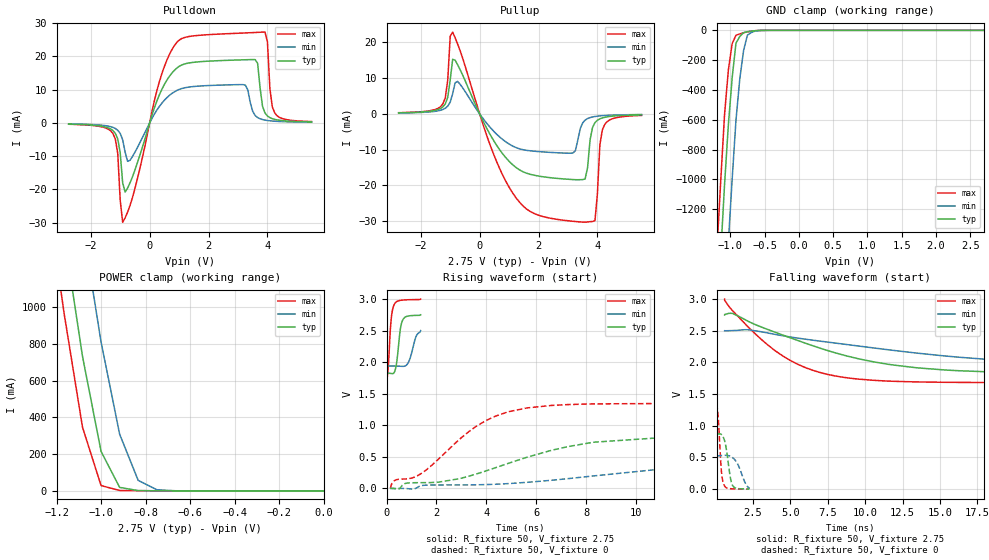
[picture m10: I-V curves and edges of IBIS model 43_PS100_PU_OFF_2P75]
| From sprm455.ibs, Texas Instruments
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|   Model Cell 43_PS100_PU_OFF_2P75
|IDG09_OUO43_PS100_PU_OFF_2P75
[Model]   43_PS100_PU_OFF_2P75
Model_type   I/O
Polarity   Non-Inverting
Enable   Active-Low
Vinl =  0.7V
Vinh =  1.7V
Cref =  15pF
Rref =  100.00M
Vref =  0V
Vmeas =  1.375
C_comp   1.5660002p   1.4978002p   1.7490998p
[Model Spec]
Vinl   0.7V   0.7V   0.7V
Vinh   1.7V   1.7V   1.7V
[Temperature Range]   25   125   -40
[Voltage Range]   2.75   2.5   3
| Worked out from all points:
|   slope of the pulldown table from 0 to 0.412 V, typ, clamps not added: 41 ohm
|   slope of the pullup table from 0 to 0.412 V, typ, clamps not added: 62.6 ohm
|   GND clamp passes 1 mA (typ) near -0.58 V on its own axis
|   POWER clamp passes 1 mA (typ) near -0.78 V on its own axis
|   rising waveform, R_fixture 50, V_fixture 2.75: 20-80 % time 161ps typ, 231ps min, 130ps max; typ from 1.82 V to 2.75 V
|   rising waveform, R_fixture 50, V_fixture 0: 20-80 % time 4.57ns typ, 8.78ns min, 2.5ns max; typ from 0 V to 0.861 V
|   falling waveform, R_fixture 50, V_fixture 2.75: 20-80 % time 7.55ns typ, 12.6ns min, 4.28ns max; typ from 2.75 V to 1.82 V
|   falling waveform, R_fixture 50, V_fixture 0: 20-80 % time 319ps typ, 552ps min, 204ps max; typ from 0.861 V to 0 V
[POWER_clamp]
|   voltage   I(typ)   I(min)   I(max)
-2.75V    16.6A      17.26A     16.24A
-1.194V   1.641A     2.388A     1.212A
-1.167V   1.399A     2.143A     971.7mA
-1.139V   1.177A     1.911A     763.3mA
-1.111V   954.8mA    1.678A     555mA
-1.083V   732.5mA    1.445A     346.6mA
-1.056V   560.1mA    1.234A     240.8mA
-1.028V   387.7mA    1.022A     135mA
-1V       215.3mA    810.7mA    29.13mA
-916.7mV  19.33mA    309.1mA    2.488mA
-833.3mV  1.75mA     57.46mA    1.352mA
0V        27.64pA    4.396nA    364.2fA
[Pulldown]
|   voltage   I(typ)   I(min)   I(max)
-2.75V    -365.9uA   -284.1uA   -404.8uA
-1.25V    -2.274mA   -1.347mA   -3.141mA
-1.083V   -4.807mA   -2.213mA   -9.196mA
-916.7mV  -18.05mA   -5.07mA    -29.89mA
-666.7mV  -18.05mA   -11.25mA   -24.87mA
333.3mV   8.511mA    4.998mA    12.5mA
1.083V    17.41mA    10.32mA    25.36mA
3.25V     19.01mA    11.37mA    27.08mA
3.583V    19.04mA    2.232mA    27.22mA
3.917V    2.992mA    841.3uA    27.33mA
4.25V     1.053mA    505.4uA    2.946mA
5.5V      292.8uA    198.8uA    397.1uA
[Pullup]
|   voltage   I(typ)   I(min)   I(max)
-2.75V    285.7uA    234.9uA    326.2uA
-1.25V    1.953mA    1.223mA    2.77mA
-1.083V   4.622mA    2.158mA    9.493mA
-916.7mV  15.25mA    5.649mA    22.87mA
-750mV    13.77mA    9.085mA    19.58mA
1.167V    -14.54mA   -9.171mA   -22.68mA
3.167V    -18.37mA   -10.95mA   -30.03mA
3.583V    -18.19mA   -1.737mA   -30.29mA
3.917V    -2.45mA    -735.4uA   -29.85mA
4.083V    -1.386mA   -565uA     -8.642mA
4.25V     -954.5uA   -457.6uA   -2.918mA
5.5V      -278.9uA   -186.4uA   -433.5uA
[GND_clamp]
|   voltage   I(typ)   I(min)   I(max)
-2.75V    -16.98A    -17.77A    -16.54A
-1.194V   -1.982A    -2.846A    -1.48A
-1.139V   -1.503A    -2.356A    -1.012A
-1.083V   -1.037A    -1.876A    -566.6mA
-1.028V   -636.6mA   -1.424A    -267.8mA
-972.2mV  -319.4mA   -999.8mA   -89.79mA
-916.7mV  -85.78mA   -603.6mA   -32.68mA
-861.1mV  -41.34mA   -325.9mA   -23.99mA
-805.6mV  -15.8mA    -135.5mA   -16.49mA
-750mV    -9.16mA    -32.45mA   -10.18mA
-638.9mV  -2.919mA   -5.132mA   -2.575mA
2.694V    26.4pA     159.6nA    263.5fA
[Ramp]
| variable   typ   min   max
dV/dt_f 0.57015078/7.6563469n 0.34585327/12.747032n 0.81281527/4.3260627n
dV/dt_r 0.52369377/4.5835117n 0.32131395/8.7485655n 0.81659858/2.5157371n
R_load = 50
[Rising Waveform]
R_fixture = 50
V_fixture = 2.75
V_fixture_min = 2.5
V_fixture_max = 3
|   time   V(typ)   V(min)   V(max)
0s        1.825V     1.939V     1.682V
69.49ps   1.825V     1.939V     1.927V
184.5ps   1.821V     1.94V      2.672V
288.7ps   1.827V     1.939V     2.896V
387.1ps   1.949V     1.938V     2.953V
545.8ps   2.502V     1.936V     2.979V
638.1ps   2.659V     1.934V     2.984V
874.2ps   2.732V     1.995V     2.989V
1.177ns   2.741V     2.401V     2.991V
1.369ns   2.75V      2.5V       3V
[Rising Waveform]
R_fixture = 50
V_fixture = 0
V_fixture_min = 0
V_fixture_max = 0
|   time   V(typ)   V(min)   V(max)
154.1ps   56.17pV    15.94nV    1.198pV
349.7ps   -5.34mV    186.5uV    131mV
807.1ps   83.49mV    -2.177mV   150.7mV
1.41ns    91.25mV    44.83mV    241.1mV
3.005ns   162.8mV    55.22mV    805.9mV
3.954ns   273.3mV    60.54mV    1.069V
5.629ns   494.5mV    96.57mV    1.275V
8.284ns   731.6mV    197.5mV    1.339V
12.39ns   841.2mV    361.7mV    1.348V
21.44ns   861.2mV    526.4mV    1.348V
[Falling Waveform]
R_fixture = 50
V_fixture = 2.75
V_fixture_min = 2.5
V_fixture_max = 3
|   time   V(typ)   V(min)   V(max)
606.5ps   2.75V      2.5V       3V
1.136ns   2.773V     2.502V     2.817V
2.246ns   2.642V     2.514V     2.545V
3.88ns    2.485V     2.447V     2.204V
5.453ns   2.35V      2.385V     1.975V
7.495ns   2.187V     2.321V     1.811V
10.58ns   2.009V     2.228V     1.718V
13.54ns   1.913V     2.145V     1.692V
18.28ns   1.851V     2.046V     1.683V
25.61ns   1.825V     1.939V     1.682V
[Falling Waveform]
R_fixture = 50
V_fixture = 0
V_fixture_min = 0
V_fixture_max = 0
|   time   V(typ)   V(min)   V(max)
65.63ps   861.2mV    526.4mV    1.348V
183.7ps   869.7mV    526.5mV    1.113V
391.3ps   862.8mV    530.5mV    286.1mV
538ps     809.3mV    533.1mV    83.23mV
692.9ps   671.5mV    534.2mV    27.13mV
971.8ps   207.3mV    521.1mV    8.013mV
1.119ns   66.22mV    500.9mV    5.787mV
1.474ns   10.33mV    397.8mV    3.395mV
1.982ns   3.339mV    99.41mV    1.848mV
2.255ns   56.17pV    15.94nV    1.198pV
